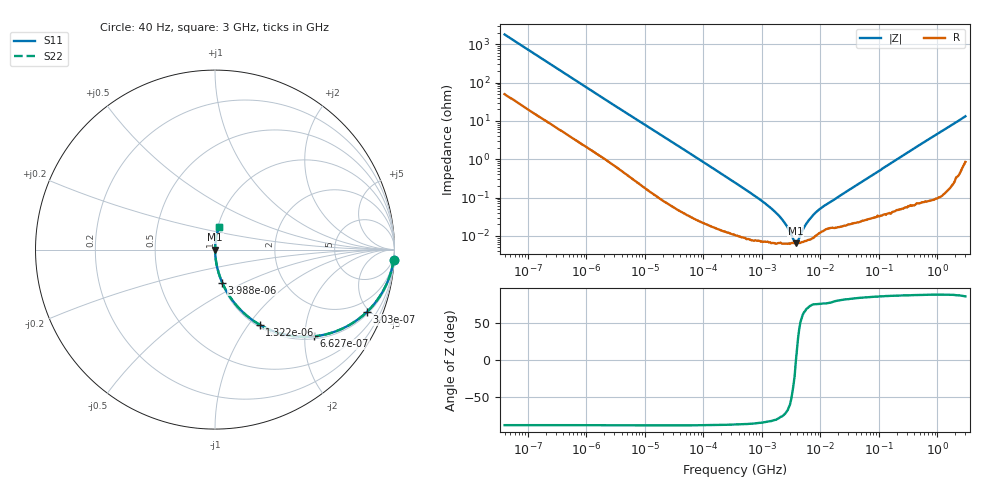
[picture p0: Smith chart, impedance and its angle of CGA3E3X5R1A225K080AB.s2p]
! S-parameter Generated by TDK Corporation
! Copyright(C) 2015 TDK Corporation.
! All Rights Reserved.
! TDK P/N: CGA3E3X5R1A225K080AB (Multilayer Ceramic Chip Capacitors)
! Property: C=2.2uF
! Size(LxWxT): 1.6x0.8x0.8mm, 0.063x0.031x0.031inches
! Model Type: s2p (Touchstone File Format Version 1.0)
! Frequency: DC=Yes Start=0.00004MHz Stop=3000MHz 396points Log-sweep
! Note: This model was converted from impedance.
! Model Generated on Jun. 23, 2015
! Hash(MD5):
! Port Assignments:
!  1 ---| |--- 2
! Applicable Conditions:
!  Temperature = 25 degC
!  DC Bias Voltage = 0 V
!  Small Signal Operation
! Terms and conditions regarding TDK Simulation Models
! (1)This simulation model is being provided solely for informational purposes. Please refer to the specifications of the products in terms of detailed characteristics of such products.
! (2)In no event shall TDK Corporation of any of its subsidiaries be liable for any loss or damage arising, directly or indirectly,
!  From any information contained in this simulation model, including, but not limited to loss or damages arising from any inaccuracies, omissions or errors in connection with such information.
! (3)Any and all copyrights on this simulation model are owned by TDK Corporation.
!  Duplication or redistribution of this simulation model without prior written permission from TDK Corporation is prohibited.
! (4)This simulation model is subject to any modification or change without any prior notice.
! (5)Neither TDK Corporation nor any of its subsidiaries shall make any warranty, express or implied,
!  Including but not limited to the correctness, implied warranties of merchantability and fitness for a particular purpose with respect to this simulation models.
! (6)The use of this simulation model shall be deemed to have consented to the terms and conditions hereof.
# MHz S MA R 50
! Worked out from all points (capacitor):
!   395 points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, 40 Hz to 3 GHz, reference 50 ohm
!   read as one part in series: C = 2.22 uF near 41.88 Hz
!   lowest |Z| = 6.45 mohm at 3.793 MHz (marker M1)
!   series resonance near 3.814 MHz, so ESL is about 780 pH
!   S11 on the Smith chart (normalised r, x): 40 Hz: 2, -36; 303 Hz: 1.13, -4.83; 662.7 Hz: 1.06, -2.23; 1.322 kHz: 1.03, -1.13; 3.988 kHz: 1.01, -0.39; 3 GHz: 1.02, +0.26
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4e-05  0.9969 -3.2  0.05565 85.2  0.05565 85.2  0.9969 -3.2
0.0001385867  0.9773 -10.8  0.1867 77.7  0.1867 77.7  0.9773 -10.8
0.0003030459  0.915 -22.3  0.3789 66.1  0.3789 66.1  0.915 -22.3
0.000662667  0.7344 -41.2  0.6587 47.2  0.6587 47.2  0.7344 -41.2
0.000834128  0.6552 -47.5  0.7375 40.9  0.7375 40.9  0.6552 -47.5
0.001321622  0.4862 -59.3  0.8604 29.1  0.8604 29.1  0.4862 -59.3
0.002192651  0.3228 -69.6  0.9377 18.8  0.9377 18.8  0.3228 -69.6
0.003988472  0.1883 -77.7  0.9773 10.8  0.9773 10.8  0.1883 -77.7
0.01739424  0.0463 -86.2  0.998 2.7  0.998 2.7  0.0463 -86.2
0.3464102  0.002445 -87.4  0.9999 0.1  0.9999 0.1  0.002445 -87.4
1.442786  0.0005214 -82.9  0.9999 0.0  0.9999 0.0  0.0005214 -82.9
1.991197  0.0003255 -78.4  0.9999 0.0  0.9999 0.0  0.0003255 -78.4
2.506407  0.0002095 -72.6  0.9999 0.0  0.9999 0.0  0.0002095 -72.6
3.303516  9.215e-05 -44.6  0.9999 0.0  0.9999 0.0  9.215e-05 -44.6
3.792615  6.446e-05 -2.1  0.9999 0.0  0.9999 0.0  6.446e-05 -2.1
4.5592  0.0001056 51.6  0.9999 -0.0  0.9999 -0.0  0.0001056 51.6
5.480732  0.0001859 66.6  0.9999 -0.0  0.9999 -0.0  0.0001859 66.6
7.22376  0.0003263 74.9  0.9999 -0.0  0.9999 -0.0  0.0003263 74.9
11.44558  0.0006002 76.7  0.9999 -0.0  0.9999 -0.0  0.0006002 76.7
150.6385  0.007425 86.5  0.9996 -0.4  0.9996 -0.4  0.007425 86.5
906.6656  0.042 86.4  0.9982 -2.4  0.9982 -2.4  0.042 86.4
3000  0.1295 78.9  0.9833 -7.4  0.9833 -7.4  0.1295 78.9
